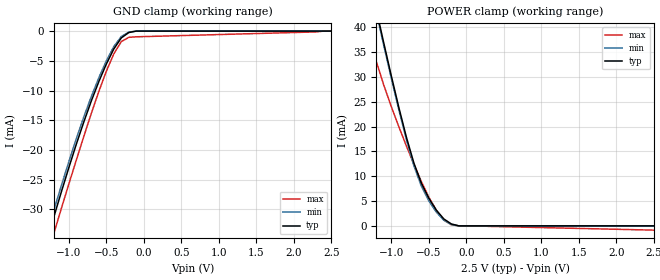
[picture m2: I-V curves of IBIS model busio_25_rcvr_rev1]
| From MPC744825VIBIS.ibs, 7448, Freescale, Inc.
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| *   BUSIO 2.5V RCVR Model Rev1.1
[Model]   busio_25_rcvr_rev1
Model_type   Input
Polarity   Non-Inverting
Vinl = 0.5V
Vinh = 1.7V
|   typ   min   max
C_comp   2.967499e-13   2.705084e-13   1.033671e-12
|   typ   min   max
[Voltage range]   2.5V   2.3V   2.7V
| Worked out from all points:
|   GND clamp passes 1 mA (typ) near -0.28 V on its own axis
|   POWER clamp passes 1 mA (typ) near -0.26 V on its own axis
[GND_clamp]
-2.7V     -100.8mA   -98.75mA   -103.3mA
-1.3V     -35.58mA   -34.37mA   -38.31mA
-1.2V     -31.27mA   -30.13mA   -34.04mA
-1.1V     -27.06mA   -25.99mA   -29.84mA
-900mV    -19.03mA   -18.1mA    -21.69mA
-700mV    -11.75mA   -11mA      -13.84mA
-600mV    -8.501mA   -7.845mA   -10.16mA
-400mV    -3.009mA   -2.605mA   -3.831mA
-300mV    -1.145mA   -910.9uA   -1.769mA
-200mV    -247.3uA   -170.3uA   -1.048mA
-100mV    0A         0A         -962.8uA
2.5V      0A         0A         0A
[POWER_clamp]
-2.7V     151.6mA    150.2mA    124.2mA
-1.4V     57.35mA    56.74mA    43.88mA
-1.3V     50.42mA    49.85mA    38.35mA
-1.2V     43.57mA    43.03mA    33.13mA
-1.1V     36.83mA    36.31mA    28.36mA
-800mV    17.94mA    17.45mA    16.15mA
-700mV    12.71mA    12.16mA    12.44mA
-600mV    8.616mA    8.017mA    8.95mA
-400mV    3.178mA    2.773mA    3.125mA
-300mV    1.399mA    1.147mA    1.166mA
-200mV    389.9uA    287uA      221.5uA
2.5V      0A         0A         -859.2uA
